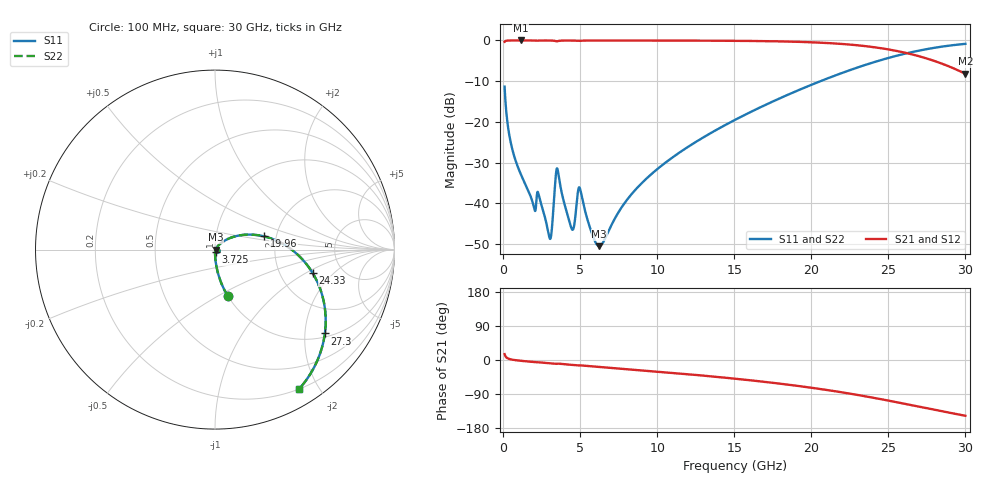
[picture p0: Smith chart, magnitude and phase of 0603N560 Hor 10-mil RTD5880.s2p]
# GHz S MA R 50
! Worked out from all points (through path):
!   3201 points, 100 MHz to 30 GHz, reference 50 ohm
!   highest |S21| = -0.01 dB at 1.156 GHz (marker M1); lowest = -8.2 dB at 30 GHz (marker M2)
!   group delay of S21, straight-line fit = 13.2 ps
!   lowest |S11| = -50.5 dB at 6.239 GHz (marker M3), VSWR 1.01, Z = 50.3 - j0.086 ohm
!   |S11| at or under -10 dB: start of sweep to 20.6 GHz
!   |S22| runs from -50.5 to -0.8 dB; largest |S21 - S12| = 0
!   S11 on the Smith chart (normalised r, x): 100 MHz: 1.00, -0.56; 3.725 GHz: 1.01, -0.03; 19.96 GHz: 1.72, +0.28; 24.33 GHz: 3.05, -1.17; 27.3 GHz: 1.10, -2.53; 30 GHz: 0.20, -1.75
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0.1  0.2706 -74.5  0.9623 15.4  0.9623 15.4  0.2706 -74.5
0.5017812  0.05533 -87.6  0.9978 1.7  0.9978 1.7  0.05533 -87.6
1.155844  0.02272 -89.5  0.9987 -2.1  0.9987 -2.1  0.02272 -89.5
1.987437  0.009198 -80.6  0.9976 -5.3  0.9976 -5.3  0.009198 -80.6
2.3425  0.01214 -77.6  0.996 -6.2  0.996 -6.2  0.01214 -77.6
3.01525  0.003779 -42.6  0.9968 -8.7  0.9968 -8.7  0.003779 -42.6
3.16475  0.004833 4.1  0.9953 -9.4  0.9953 -9.4  0.004833 4.1
3.46375  0.02575 -14.2  0.9743 -10.1  0.9743 -10.1  0.02575 -14.2
3.725375  0.01617 -71.7  0.9921 -10.1  0.9921 -10.1  0.01617 -71.7
4.472875  0.004811 -45.3  0.9959 -13.0  0.9959 -13.0  0.004811 -45.3
4.893344  0.01516 -25.3  0.9851 -14.2  0.9851 -14.2  0.01516 -25.3
5.089563  0.01265 -62.5  0.9914 -14.4  0.9914 -14.4  0.01265 -62.5
6.238844  0.002992 -16.6  0.9969 -18.3  0.9969 -18.3  0.002992 -16.6
8.042188  0.01108 49.2  0.9966 -24.1  0.9966 -24.1  0.01108 49.2
10.06978  0.02697 51.3  0.9958 -30.8  0.9958 -30.8  0.02697 51.3
15.05  0.106 37.6  0.9884 -49.3  0.9884 -49.3  0.106 37.6
19.95547  0.2827 15.1  0.9493 -72.9  0.9493 -72.9  0.2827 15.1
20.03956  0.287 14.7  0.948 -73.4  0.948 -73.4  0.287 14.7
24.32834  0.5598 -13.5  0.8124 -101.9  0.8124 -101.9  0.5598 -13.5
25.01978  0.6105 -18.9  0.7745 -107.2  0.7745 -107.2  0.6105 -18.9
27.29966  0.77 -37.3  0.6156 -125.7  0.6156 -125.7  0.77 -37.3
30  0.9077 -59.1  0.3893 -147.1  0.3893 -147.1  0.9077 -59.1
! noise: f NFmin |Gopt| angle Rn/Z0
0.1  0.0002927  0.9186  0.3523  0.0007941
3.417  0.01259  0.9349  10.03  0.04275
6.743  0.006616  0.7768  19.72  0.005888
10.06  0.009  0.7598  29.2  0.007118
13.39  0.01192  0.7615  38.48  0.009056
16.7  0.01559  0.774  47.48  0.01184
20.03  0.02058  0.7956  56.24  0.01625
23.35  0.02803  0.8254  64.75  0.02416
26.67  0.0408  0.8629  73.09  0.04131
30  0.06804  0.9074  81.32  0.09302
